FUNCTION F_ADD_LIN_NODE_PARITY : BYTE
VAR_INPUT
   nNodeID:BYTE;  // Inputvariable: node-Id
   nReqLen:BYTE;  // Inputvariable: length-identification: 2,4,8 Byte-Frame
END_VAR
VAR
   bParity0:BYTE; // Internal intermediate value parity 0
   bParity1:BYTE; // Internal intermediate value parity 1
   nPrepId:BYTE;  // Intermediate value for PID
END_VAR

nPrepId := nNodeID OR SHL(nReqLen,4);

bParity0 :=
(nNodeID AND 2#0001)
XOR (SHR((nNodeID AND 2#0010), 1))
XOR (SHR((nNodeID AND 2#0100), 2))
XOR (SHR((nNodeID AND 2#0001_0000), 4));

bParity1 := 16#01 AND (NOT(
SHR((nNodeID AND 2#0010), 1)
XOR (SHR((nNodeID AND 2#1000),3))
XOR (SHR((nNodeID AND 2#0001_0000), 4))
XOR (SHR((nNodeID AND 2#0010_0000), 5))));

F_ADD_LIN_NODE_PARITY := nPrepId OR SHL(bParity0,6) OR SHL(bParity1,7);

END_FUNCTION
